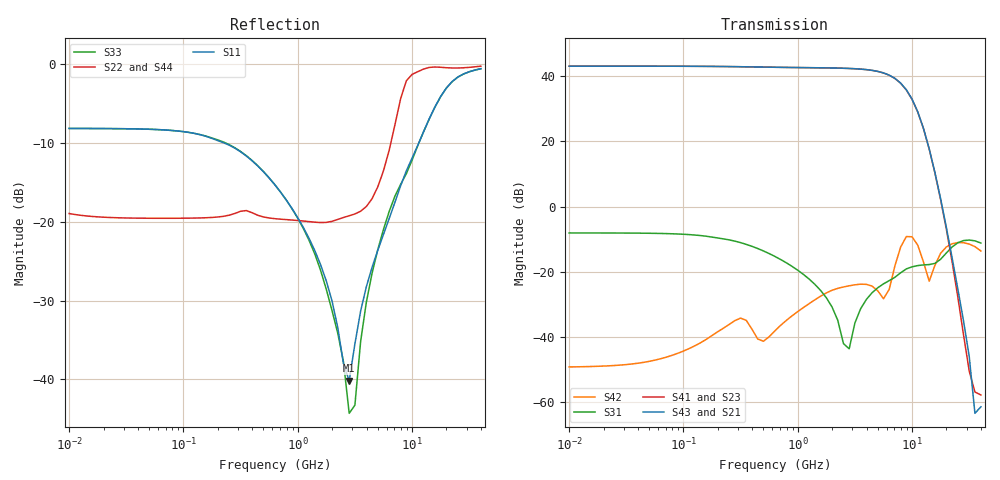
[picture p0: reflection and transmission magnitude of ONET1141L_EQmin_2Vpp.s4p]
! Touchstone Ver. 1.0
! Fri Mar 23 19:27:27 2012
! Number of ports is 4
# Hz	S	DB	R	50.000000
! SCATTERING PARAMETERS  :
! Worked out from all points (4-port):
!   73 points, 10 MHz to 40 GHz, reference 50 ohm
!   strongest paths, dB at 10 MHz, 79.43 MHz, 631 MHz, 5.012 GHz, 40 GHz:
!     S43: 43.0, 43.0, 42.7, 41.4, -61.4
!     S41: 43.0, 43.0, 42.7, 41.4, -57.7
!     S23: 43.0, 43.0, 42.7, 41.4, -57.8
!     S21: 43.0, 43.0, 42.7, 41.4, -61.5
!     S31: -8.1, -8.3, -15.3, -24.9, -11.2
!     S42: -49.1, -45.6, -38.1, -25.8, -13.6
!   lowest |S11| = -40.2 dB at 2.818 GHz (marker M1), VSWR 1.02, Z = 49.1 + j0.33 ohm
!   |S11| at or under -10 dB: 229.2 MHz to 11.43 GHz (11.21 GHz wide, 192 % of centre)
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1e7  -8.13 -2.0  -109.36 92.2  -8.07 -1.7  -108.83 92.7
     43.03 -177.8  -18.93 24.6  43.03 2.2  -49.47 12.9
     -8.07 -1.7  -109.15 92.1  -8.13 -2.0  -109.01 93.7
     43.04 2.2  -49.13 12.7  43.04 -177.8  -18.92 24.6
7.079458e8  -16.22 -71.3  -54.43 96.9  -16.20 -70.4  -54.45 96.8
            42.67 147.9  -19.65 -16.1  42.67 -32.1  -37.18 70.4
            -16.20 -70.3  -54.42 96.8  -16.21 -71.5  -54.43 96.8
            42.68 -32.0  -36.39 67.6  42.68 148.0  -19.58 -15.4
2.818383e9  -40.16 160.0  -43.86 -6.1  -48.11 -50.3  -43.86 -6.2
            42.32 55.9  -19.22 -62.9  42.32 -124.1  -23.65 37.3
            -43.58 126.6  -43.84 -6.2  -44.30 -118.5  -43.85 -6.1
            42.33 -123.9  -24.27 36.4  42.34 56.1  -19.09 -65.0
3.981072e9  -28.24 93.2  -45.49 -29.3  -31.00 88.1  -45.49 -29.4
            41.96 3.3  -18.04 -105.3  41.95 -176.9  -23.74 15.9
            -28.46 78.0  -45.48 -29.4  -30.20 107.6  -45.49 -29.2
            41.97 -176.4  -23.82 15.3  41.99 3.5  -18.01 -105.4
5.623413e9  -21.58 80.0  -45.71 -45.7  -23.11 74.8  -45.69 -46.0
            40.94 -73.8  -13.50 -161.6  40.92 105.9  -28.69 -45.4
            -23.67 65.0  -45.71 -45.7  -20.94 87.0  -45.72 -45.4
            40.96 106.5  -28.24 -62.1  40.98 -73.5  -13.13 -160.4
8.912509e9  -13.51 56.1  -42.80 -107.0  -19.68 51.5  -42.74 -107.3
            35.68 126.7  -2.08 98.5  35.57 -54.0  -9.36 87.8
            -19.09 55.8  -42.62 -107.1  -13.87 54.1  -42.65 -106.8
            35.74 -53.5  -9.18 87.1  35.81 126.7  -2.02 98.0
4e10  -0.54 -107.5  -58.84 2.1  -11.16 -16.5  -58.58 1.1
      -61.50 29.3  -0.22 -118.6  -57.83 12.8  -13.60 -28.1
      -11.16 -16.5  -58.67 1.5  -0.54 -107.4  -58.69 1.8
      -57.73 12.3  -13.60 -28.1  -61.36 28.2  -0.22 -118.6
